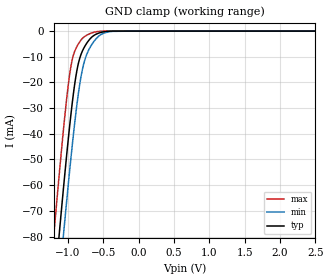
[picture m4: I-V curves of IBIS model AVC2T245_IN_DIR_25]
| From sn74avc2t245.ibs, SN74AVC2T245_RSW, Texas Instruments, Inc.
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[Model]   AVC2T245_IN_DIR_25
Model_type  Input
Vinl=0.7
Vinh=1.6
| variable   typ   min   max
C_comp   1.98pF   1.61pF   2.53pF
[Temperature Range]   40   100   -40
| Ambient temperature   25   85   -40
[Voltage range]   2.5   2.3   2.7
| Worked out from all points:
|   GND clamp passes 1 mA (typ) near -0.58 V on its own axis
[GND Clamp]
| AVC2T245_IN_DIR_25
|   Voltage   I(typ)   I(min)   I(max)
-4.6V     -1.266A    -1.277A    -1.254A
-1.215V   -107.3mA   -125.7mA   -84.13mA
-1.19V    -99.51mA   -117.9mA   -76.26mA
-1.13V    -81mA      -99.35mA   -57.75mA
-1.11V    -74.94mA   -93.26mA   -51.76mA
-1.06V    -60.14mA   -78.3mA    -37.34mA
-960mV    -32.94mA   -49.96mA   -14.03mA
-855mV    -12.87mA   -24.8mA    -5.101mA
-755mV    -5.619mA   -10.66mA   -1.918mA
-565mV    -793.5uA   -1.982mA   -117.3uA
-365mV    -13.86uA   -100.1uA   -144.9nA
2.5V      156.4pA    16.88nA    32.51pA
